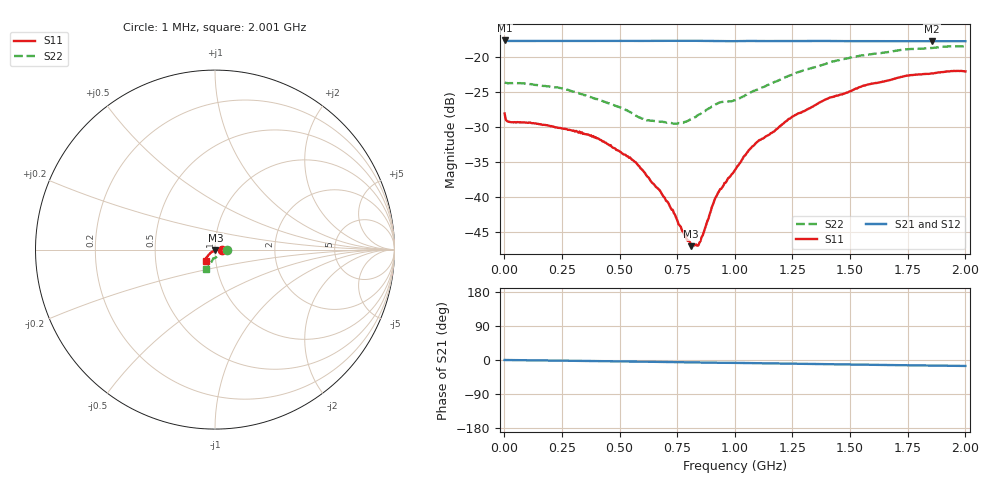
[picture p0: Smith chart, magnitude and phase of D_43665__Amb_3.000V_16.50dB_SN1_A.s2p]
! device id: 43665_
! dir: \\malibu\benchdata\1_engineers\tn_data\43665_75ohm\new\sparar\43665_\amb\3p000v\16p50db
! Serial: 1
! Insertion: A
! Temp: Amb
! VDD: 3.000V
! Attenuation Step: 16.50dB
! IDD: 1.447804e+00mA
! FILE NAME
! DATE 03-27-2009 08:37:24
! CORRECTED  DATA
#  Hz  S  RI  R  75
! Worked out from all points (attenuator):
!   401 points, 1 MHz to 2.001 GHz, reference 75 ohm
!   highest |S21| = -17.56 dB at 1 MHz (marker M1); lowest = -17.7 dB at 1.856 GHz (marker M2)
!   lowest |S11| = -47.1 dB at 811 MHz (marker M3), VSWR 1.01, Z = 75.4 - j0.557 ohm
!   |S11| at or under -10 dB: start of sweep to end of sweep
!   |S22| runs from -29.5 to -18.4 dB; largest |S21 - S12| = 0.00084
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1000000  0.0397 -0.000448  0.1325 -2.37e-05  0.1317 -0.000244  0.0662 -0.000694
2.6e7  0.0344 6.45e-05  0.1314 -0.000406  0.1314 -0.00043  0.0655 -0.000444
2.36e8  0.0312 0.00183  0.1314 -0.00379  0.1315 -0.00374  0.0606 -0.0023
3.36e8  0.029 0.00202  0.1314 -0.00548  0.1314 -0.00539  0.0544 -0.0042
4.06e8  0.0262 0.00272  0.1314 -0.00656  0.1314 -0.00651  0.0495 -0.0069
5.46e8  0.0191 0.00147  0.1313 -0.00924  0.1313 -0.00911  0.0382 -0.0137
5.96e8  0.0158 0.000947  0.1311 -0.0101  0.1312 -0.00996  0.0328 -0.0161
6.71e8  0.0113 -0.000617  0.1311 -0.0114  0.1312 -0.0112  0.0271 -0.0217
7.46e8  0.00669 -0.0022  0.1311 -0.0129  0.1312 -0.0127  0.0202 -0.0268
7.86e8  0.00417 -0.00313  0.131 -0.0138  0.131 -0.0136  0.0161 -0.0305
8.11e8  0.00244 -0.00369  0.1309 -0.0143  0.131 -0.0141  0.0135 -0.0335
8.46e8  0.000195 -0.00465  0.1308 -0.015  0.1309 -0.0148  0.0104 -0.0377
9.21e8  -0.00629 -0.00795  0.13 -0.0166  0.1301 -0.0163  0.00135 -0.0464
1.001e9  -0.0115 -0.0105  0.1299 -0.0173  0.13 -0.017  -0.00909 -0.0484
1.051e9  -0.0166 -0.0121  0.1301 -0.0184  0.1302 -0.0181  -0.0111 -0.0528
1.101e9  -0.0198 -0.0154  0.1298 -0.0196  0.13 -0.0192  -0.0134 -0.0577
1.241e9  -0.0289 -0.0224  0.1294 -0.0222  0.1297 -0.0218  -0.0219 -0.0713
1.336e9  -0.0342 -0.0281  0.1291 -0.0239  0.1295 -0.0236  -0.0276 -0.0796
1.551e9  -0.0456 -0.0421  0.128 -0.028  0.1285 -0.0279  -0.0377 -0.0965
1.671e9  -0.0489 -0.0483  0.1274 -0.0301  0.1278 -0.0301  -0.0418 -0.1014
1.856e9  -0.0507 -0.0579  0.1265 -0.0331  0.1266 -0.0331  -0.0474 -0.107
2.001e9  -0.0499 -0.0619  0.126 -0.0354  0.126 -0.0357  -0.051 -0.1085
